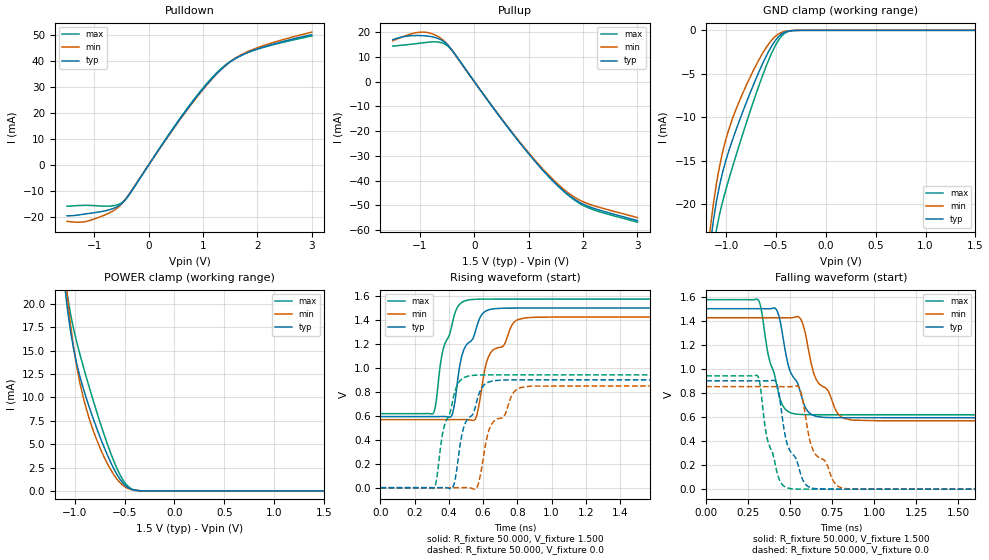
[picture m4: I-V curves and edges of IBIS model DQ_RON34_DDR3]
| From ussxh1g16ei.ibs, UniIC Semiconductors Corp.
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|   Model DQ_RON34_DDR3
[Model] DQ_RON34_DDR3
Model_type I/O
Vinl =  0.615V
Vinh =  0.885V
Vmeas =  0.750V
Rref =  50.000
Vref =  0.750V
C_comp   1.232pF   1.219pF   1.235pF
[Model Spec]
Vinh   0.885V   0.847V   0.922V
Vinl   0.615V   0.577V   0.652V
Vmeas   0.750V   0.712V   0.787V
Vref   0.750V   0.712V   0.787V
Rref   50.000   NA   NA
[Temperature Range]   25.000   95.000   -40.000
[Voltage Range]   1.500V   1.425V   1.575V
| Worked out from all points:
|   slope of the pulldown table from 0 to 0.225 V, typ, clamps not added: 31.9 ohm
|   slope of the pullup table from 0 to 0.225 V, typ, clamps not added: 32.6 ohm
|   GND clamp passes 1 mA (typ) near -0.49 V on its own axis
|   POWER clamp passes 1 mA (typ) near -0.53 V on its own axis
|   rising waveform, R_fixture 50.000, V_fixture 1.500: 20-80 % time 117ps typ, 158ps min, 88.7ps max; typ from 0.594 V to 1.5 V
|   rising waveform, R_fixture 50.000, V_fixture 0.0: 20-80 % time 114ps typ, 153ps min, 87.5ps max; typ from 0 V to 0.9 V
|   falling waveform, R_fixture 50.000, V_fixture 1.500: 20-80 % time 116ps typ, 152ps min, 88.3ps max; typ from 1.5 V to 0.594 V
|   falling waveform, R_fixture 50.000, V_fixture 0.0: 20-80 % time 110ps typ, 146ps min, 82.4ps max; typ from 0.9 V to 0 V
[Pulldown]
|Voltage   I(typ)   I(min)   I(max)
-1.5V     -19.49mA   -21.6mA    -15.82mA
-1.086V   -18.54mA   -21.29mA   -15.49mA
-718mV    -17.14mA   -18.33mA   -15.75mA
-488mV    -14.63mA   -14.76mA   -14.41mA
-350mV    -11.06mA   -10.9mA    -11.21mA
294mV     9.184mA    9.034mA    9.338mA
754mV     22.67mA    22.4mA     23mA
1.076V    31.08mA    30.86mA    31.43mA
1.352V    37.06mA    37.01mA    37.34mA
1.582V    40.65mA    40.82mA    40.81mA
1.904V    43.84mA    44.25mA    43.81mA
3V        50.02mA    51.01mA    49.51mA
[Pullup]
|Voltage   I(typ)   I(min)   I(max)
-1.5V     16.95mA    16.48mA    14.34mA
-1.14V    18.56mA    19.4mA     15.15mA
-910mV    18.5mA     19.96mA    15.76mA
-680mV    17.52mA    18.39mA    16.02mA
-496mV    14.97mA    15.06mA    14.51mA
-358mV    11.17mA    11.1mA     11.02mA
746mV     -22.19mA   -21.92mA   -22.05mA
1.16V     -33.28mA   -32.84mA   -33.19mA
1.528V    -41.84mA   -41.22mA   -41.89mA
1.804V    -46.92mA   -46.11mA   -47.2mA
2.034V    -49.79mA   -48.8mA    -50.32mA
3V        -56.11mA   -54.9mA    -56.74mA
[GND_clamp]
|Voltage   I(typ)   I(min)   I(max)
-1.5V     -77.15mA   -73.99mA   -84.26mA
-1.159V   -24.58mA   -22.75mA   -27.74mA
-1.128V   -21.88mA   -19.96mA   -25.03mA
-1.097V   -19.64mA   -17.59mA   -22.88mA
-1.066V   -17.82mA   -15.61mA   -21.14mA
-1.004V   -15mA      -12.58mA   -18.36mA
-880mV    -10.79mA   -8.48mA    -13.61mA
-632mV    -3.776mA   -2.594mA   -5.119mA
-477mV    -756.2uA   -431.9uA   -1.164mA
-415mV    -225.6uA   -131.2uA   -354.1uA
-322mV    -19.15uA   -14.82uA   -24.1uA
1.5V      0A         0A         0A
[POWER_clamp]
|Voltage   I(typ)   I(min)   I(max)
-1.5V     91.1mA     92.64mA    94.46mA
-1.104V   22.28mA    23.97mA    23.43mA
-1.073V   19.41mA    20.63mA    20.89mA
-1.042V   17.07mA    17.76mA    18.91mA
-980mV    13.62mA    13.3mA     15.93mA
-918mV    11.11mA    10.16mA    13.45mA
-856mV    9.013mA    7.787mA    11.15mA
-670mV    3.78mA     2.864mA    4.931mA
-577mV    1.775mA    1.269mA    2.414mA
-484mV    502.3uA    362.1uA    693.5uA
-329mV    12.96uA    15.92uA    9.805uA
1.5V      0A         0A         0A
[Ramp]
| variable   typ   min   max
dV/dt_r   0.540/0.114n   0.511/0.153n   0.565/87.402p
dV/dt_f   0.544/0.116n   0.514/0.152n   0.574/88.209p
R_load = 50.000
[Rising Waveform]
R_fixture= 50.000
V_fixture= 1.500
V_fixture_min= 1.425
V_fixture_max= 1.575
|time   V(typ)   V(min)   V(max)
0s        593.7mV    568.1mV    618.6mV
312ps     593.7mV    568.1mV    626.8mV
361ps     594.3mV    568.1mV    1.122V
418ps     605.9mV    568.1mV    1.36V
470ps     1.068V     568.4mV    1.541V
504ps     1.195V     568.6mV    1.564V
561ps     1.336V     594.2mV    1.573V
642ps     1.489V     1.123V     1.575V
841ps     1.5V       1.418V     1.575V
3ns       1.5V       1.425V     1.575V
[Rising Waveform]
R_fixture= 50.000
V_fixture= 0.0
V_fixture_min= 0.0
V_fixture_max= 0.0
|time   V(typ)   V(min)   V(max)
0s        129.7nV    526.6nV    54.76nV
313ps     -14.98uV   12.17uV    -1.442mV
368ps     915.5uV    29.06uV    486.6mV
421ps     -1.313mV   -14uV      718.8mV
510ps     575.1mV    1.028mV    930.6mV
568ps     749mV      15.89mV    940.2mV
611ps     864.8mV    337.8mV    941.6mV
647ps     888.4mV    524.2mV    941.9mV
819ps     900.3mV    835.9mV    942.1mV
3ns       900.5mV    852mV      942.1mV
[Falling Waveform]
R_fixture= 50.000
V_fixture= 1.500
V_fixture_min= 1.425
V_fixture_max= 1.575
|time   V(typ)   V(min)   V(max)
0s        1.5V       1.425V     1.575V
307ps     1.5V       1.425V     1.577V
419ps     1.49V      1.425V     870.1mV
454ps     1.289V     1.425V     699.3mV
517ps     933.4mV    1.426V     629mV
568ps     767.4mV    1.398V     620.6mV
615ps     632.4mV    1.112V     619mV
653ps     606.5mV    916.6mV    618.7mV
820ps     593.9mV    588.4mV    618.6mV
3ns       593.7mV    568.1mV    618.6mV
[Falling Waveform]
R_fixture= 50.000
V_fixture= 0.0
V_fixture_min= 0.0
V_fixture_max= 0.0
|time   V(typ)   V(min)   V(max)
0s        900.5mV    852mV      942.1mV
306ps     900.4mV    852mV      941.3mV
357ps     899.9mV    852mV      460.8mV
419ps     877.9mV    852mV      151.7mV
494ps     331.2mV    851.4mV    6.577mV
557ps     149.4mV    834.7mV    442.5uV
602ps     26.31mV    509.6mV    61.49uV
642ps     5.371mV    305.4mV    11.94uV
799ps     10.09uV    13.61mV    304.3nV
3ns       160.5nV    586.1nV    216.9nV
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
